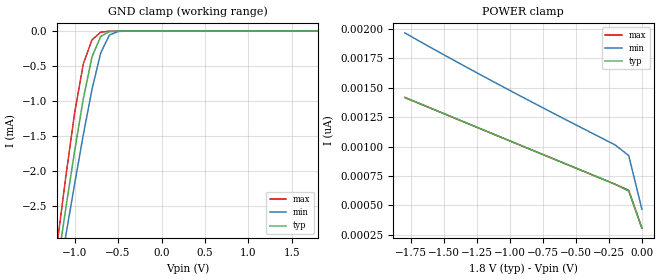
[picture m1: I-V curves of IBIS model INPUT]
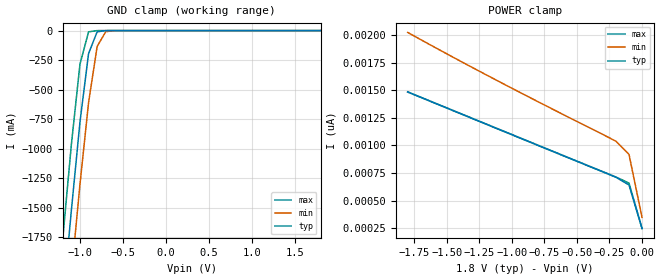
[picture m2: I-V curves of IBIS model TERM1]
|   PERICOM SEMICONDUCTOR CORP
|   IBIS Model of PI3CH480
|   Product Family: 3CH
|   TSSOP (L) Package
[IBIS Ver] 3.2
[Comment char] |_char
[File Name] pi3ch480_l_18v.ibs
[File Rev] 1.0
[Source] File originated at Pericom Semiconductor Corp.
[Date] 11/20/15
[Disclaimer] (C) Copyright PERICOM Semiconductor Corporation
   All rights reserved
  Pericom Semiconductor Corporation hereby grants the user of
  this IBIS model a non-exclusive, nontransferable license to
  use this IBIS model under the following terms.
  This IBIS model is provided on an "AS IS" basis and Pericom
  makes absolutely no warranty with respect to the information
  contained herein. PERICOM DISCLAIMS AND CUSTOMER WAIVES ALL
  WARRANTIES, EXPRESSED OR IMPLIED, INCLUDING WARRANTIES OF
  MERCHANTABILITY OR FITNESS FOR A PARTICULAR PURPOSE. The
  entire risk as to quality and performance is with the customer.
  Accordingly, in no event shall the company be liable for any
  damages, whether in contract or tort, including any lost
  profits or other incidental, consequential, exemplary, or
  punitive damages arising out of the use or application of the
  IBIS model provided in this package. Further, Pericom reserves
  the right to make changes without notice to any product herein
  to improve reliability, function, or design. Pericom does not
  convey any license under patent rights or any other intellectual
  property rights, including those of third parties.
  The user is granted this license only to use the IBIS model
  and is not granted rights to sell, load, rent, lease or license
  the IBIS model in whole or in part, or in modified form to anyone
  other than user. User may modify the IBIS model to suit its specific
  application but rights to derivative works and such modifications
  shall belong to Pericom.
  Pericom is not obligated to provide maintenance or support
  for the licensed IBIS model.
  Contact Pericom at ATTN: APPLICATION ENGINEERING / IBIS MODELS
  1545 Barber Lane Milpitas, CA 95035 USA.
[Component] PI3CH480
[Manufacturer] Pericom Semiconductor Corp.
[Package]
| variable   typ   min   max
R_pkg   0.05122ohm   0.05070ohm   0.05174ohm
L_pkg   2.82616nH   2.45517nH   3.19714nH
C_pkg   0.42513pF   0.33872pF   0.51154pF
[Pin]   signal_name   model_name   R_pin   L_pin   C_pin
1   S   INPUT   0.05174   3.19714nH   0.51154pF
2   IA0   TERM1   0.05140   2.94981nH   0.45394pF
3   IA1   TERM1   0.05105   2.70250nH   0.39633pF
4   YA   TERM2   0.05070   2.45517nH   0.33872pF
5   IB0   TERM1   0.05070   2.45517nH   0.33872pF
6   IB1   TERM1   0.05105   2.70250nH   0.39633pF
7   YB   TERM2   0.05140   2.94981nH   0.45394pF
8   GND   GND   0.05174   3.19714nH   0.51154pF
9   YC   TERM2   0.05174   3.19714nH   0.51154pF
10   IC1   TERM1   0.05140   2.94981nH   0.45394pF
11   IC0   TERM1   0.05105   2.70250nH   0.39633pF
12   YD   TERM2   0.05070   2.45517nH   0.33872pF
13   ID1   TERM1   0.05070   2.45517nH   0.33872pF
14   ID0   TERM1   0.05105   2.70250nH   0.39633pF
15   _EN   INPUT   0.05140   2.94981nH   0.45394pF
16   VCC   POWER   0.05174   3.19714nH   0.51154pF
[Series Switch Groups]
On 1 /
Off 2 /
[Series Pin Mapping]   pin_2   model_name  function_table_group
2   4   SWITCH1   1
5   7   SWITCH1   1
11   9   SWITCH1   1
14   12   SWITCH1   1
3   4   SWITCH1   2
6   7   SWITCH1   2
10   9   SWITCH1   2
13   12   SWITCH1   2
|   Model SWITCH1
[Model] SWITCH1
Model_type Series_switch
| variable   typ   min   max
C_comp   6.40pF   6.30pF   6.50pF
[Voltage Range]   1.800V   1.620V   1.980V
[GND Clamp Reference]   0.000V   0.000V   0.000V
[POWER Clamp Reference]   1.800V   1.620V   1.980V
[On]
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[OFF]
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| Models and submodels in the file (4): INPUT (Input), SWITCH1 (Series_switch), TERM1 (Terminator), TERM2 (Terminator)
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|   Model INPUT
[Model] INPUT
Model_type Input
Vinl = 0.600V
Vinh = 1.200V
| variable   typ   min   max
C_comp   1.800pF   1.700pF   1.900pF
[Voltage Range]   1.800V   1.620V   1.980V
[GND Clamp Reference]   0.000V   0.000V   0.000V
[POWER Clamp Reference]   1.800V   1.620V   1.980V
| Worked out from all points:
|   GND clamp passes 1 mA (typ) near -0.90 V on its own axis
[GND Clamp]
| Voltage   I(typ)   I(min)   I(max)
-1.8V     -8.577mA   -8.286mA   -9.176mA
-1.2V     -3.364mA   -3.668mA   -3.042mA
-1.1V     -2.528mA   -2.921mA   -2.075mA
-1V       -1.72mA    -2.189mA   -1.175mA
-900mV    -970.6uA   -1.485mA   -470.9uA
-800mV    -370.2uA   -835.9uA   -124.8uA
-700mV    -77.27uA   -313.6uA   -15.69uA
-600mV    -8.132uA   -56.97uA   -899.1nA
-500mV    -581.9nA   -5.514uA   -27.4nA
1.8V      304.9pA    998.4pA    16.08pA
[POWER Clamp]   |Note: Vtable = Vcc - Voutput
| Voltage   I(typ)   I(min)   I(max)
-1.8V     1.418nA    1.968nA    1.417nA
-1.1V     1.093nA    1.536nA    1.093nA
-200mV    677.5pA    1.011nA    677pA
-100mV    620.2pA    922.6pA    627.1pA
0V        304.9pA    464.9pA    304.7pA
|   Model TERM1
[Model] TERM1
Model_type Terminator
| variable   typ   min   max
C_comp   3.200pF   3.150pF   3.350pF
[Voltage Range]   1.800V   1.620V   1.980V
[GND Clamp Reference]   0.000V   0.000V   0.000V
[POWER Clamp Reference]   1.800V   1.620V   1.980V
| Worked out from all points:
|   GND clamp passes 1 mA (typ) near -0.71 V on its own axis
[GND Clamp]
| Voltage   I(typ)   I(min)   I(max)
-1.8V     -7.058A    -7.466A    -6.642A
-1.2V     -2.312A    -2.839A    -1.76A
-1.1V     -1.522A    -2.068A    -964.6mA
-1V       -774.2mA   -1.302A    -284.3mA
-900mV    -194.8mA   -609.8mA   -10.79mA
-800mV    -10.29mA   -134.3mA   -176uA
-700mV    -369.5uA   -9.267mA   -1.644uA
-500mV    -244.1nA   -27.85uA   -123.6pA
1.8V      244.8pA    1.023nA    53.58pA
[POWER Clamp]   |Note: Vtable = Vcc - Voutput
| Voltage   I(typ)   I(min)  I(max)
-1.8V     1.483nA    2.023nA    1.485nA
-1.1V     1.144nA    1.579nA    1.147nA
-200mV    710.2pA    1.037nA    713pA
-100mV    640.5pA    917.3pA    657.4pA
0V        244.8pA    347.1pA    248.7pA
